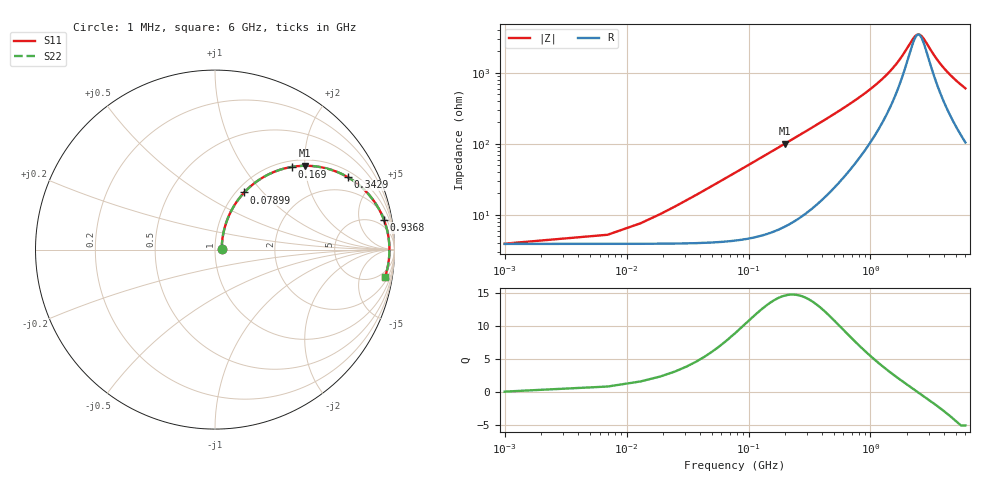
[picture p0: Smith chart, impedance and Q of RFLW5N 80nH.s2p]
!Vishay Electro-Films
!RFLW5N8000B - 80 nH Spiral Inductor on Quartz
!Measured in series configuration
!May 2011
# GHz S MA R 50
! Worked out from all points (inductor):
!   1001 points, 1 MHz to 6 GHz, reference 50 ohm
!   read as one part in series: L = 79.8 nH near 31 MHz
!   highest Q = 14.7 at 199 MHz (marker M1), where L = 80.3 nH
!   self-resonance near 2.468 GHz
!   S11 on the Smith chart (normalised r, x): 1 MHz: 1.08, +0.01; 78.99 MHz: 1.09, +0.79; 169 MHz: 1.12, +1.70; 342.9 MHz: 1.26, +3.50; 936.8 MHz: 3, +11; 6 GHz: 3, -12
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0.001  0.03781 7.1  0.9625 -0.3  0.9625 -0.3  0.03781 7.1
0.048992  0.233 67.3  0.9352 -13.3  0.9352 -13.3  0.233 67.3
0.06099  0.2845 65.9  0.9211 -16.4  0.9211 -16.4  0.2845 65.9
0.078987  0.3573 62.9  0.8958 -20.8  0.8958 -20.8  0.3573 62.9
0.12098  0.5029 55.2  0.8243 -30.1  0.8243 -30.1  0.5029 55.2
0.168972  0.6275 47.2  0.7357 -38.8  0.7357 -38.8  0.6275 47.2
0.198967  0.6863 42.9  0.6823 -43.2  0.6823 -43.2  0.6863 42.9
0.264956  0.7777 35.2  0.578 -50.9  0.578 -50.9  0.7777 35.2
0.342943  0.8426 28.6  0.4804 -57.2  0.4804 -57.2  0.8426 28.6
0.438927  0.8884 22.9  0.3912 -62.3  0.3912 -62.3  0.8884 22.9
0.564906  0.9209 17.9  0.3088 -66.4  0.3088 -66.4  0.9209 17.9
0.936844  0.9558 10.0  0.1761 -70.5  0.1761 -70.5  0.9558 10.0
1.00283  0.9585 9.1  0.1613 -70.6  0.1613 -70.6  0.9585 9.1
2.00467  0.9713 1.9  0.04319 -47.5  0.04319 -47.5  0.9713 1.9
2.26862  0.9719 0.8  0.031 -24.4  0.031 -24.4  0.9719 0.8
2.46059  0.972 0.0  0.02802 -0.9  0.02802 -0.9  0.972 0.0
2.65256  0.972 -0.6  0.03019 21.4  0.03019 21.4  0.972 -0.6
3.0005  0.9716 -1.8  0.0416 46.1  0.0416 46.1  0.9716 -1.8
3.46842  0.9707 -3.1  0.06105 59.7  0.06105 59.7  0.9707 -3.1
4.00233  0.9691 -4.5  0.08333 66.0  0.08333 66.0  0.9691 -4.5
5.00417  0.9652 -6.9  0.1226 70.1  0.1226 70.1  0.9652 -6.9
6  0.9602 -9.0  0.1588 71.0  0.1588 71.0  0.9602 -9.0
